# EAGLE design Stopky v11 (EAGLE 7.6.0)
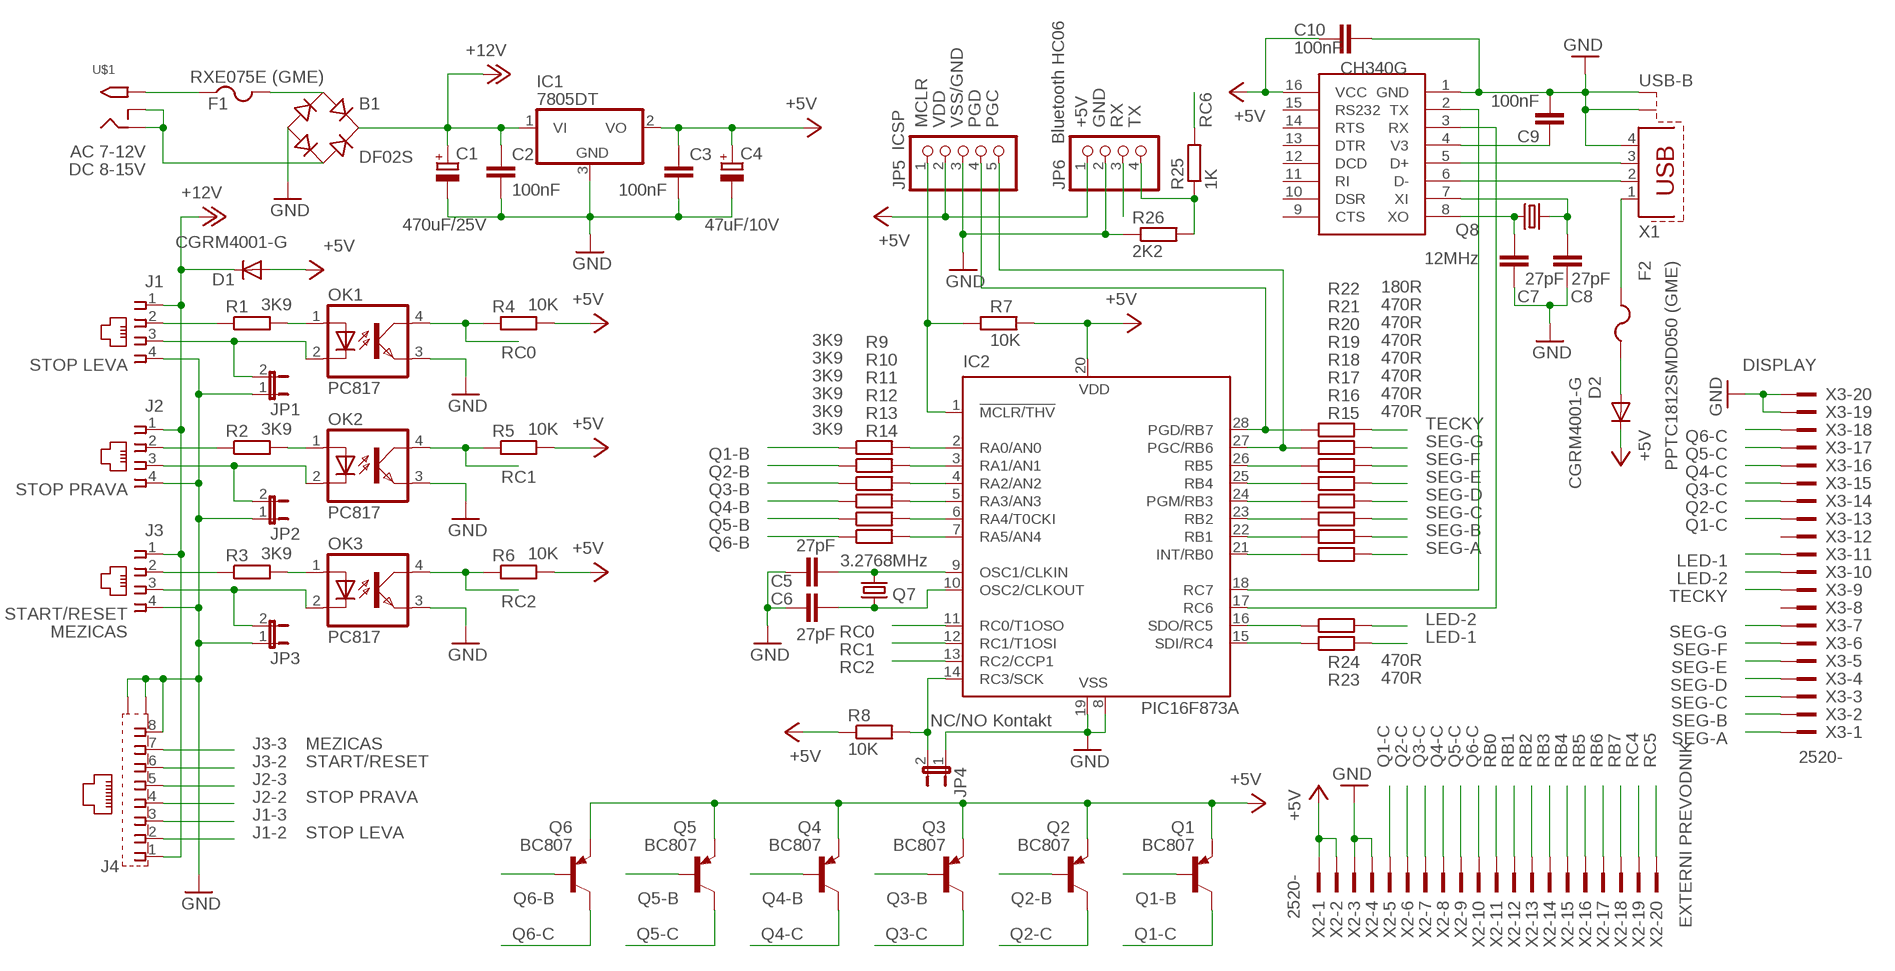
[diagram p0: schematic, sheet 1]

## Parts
B1  DF02S  [DFS]
C1  470uF/25V  CPOL-EUE3.5-10  [E3,5-10]
C2  100nF  C-EUC1206  [C1206]
C3  100nF  C-EUC1206  [C1206]
C4  47uF/10V  CPOL-EUSMCC  [SMC_C]
C5  27pF  C-EUC1206  [C1206]
C6  27pF  C-EUC1206  [C1206]
C7  27pF  C-EUC1206  [C1206]
C8  27pF  C-EUC1206  [C1206]
C9  100nF  C-EUC1206  [C1206]
C10  100nF  C-EUC1206  [C1206]
D1  CGRM4001-G  [SOD-123_MINI-SMA]
D2  CGRM4001-G  [SOD-123_MINI-SMA]
F1  RXE075E (GME)  PTCFUSE-1812  [1812]
F2  PPTC1812SMD050 (GME)  PTCFUSE-1812  [1812]
IC1  7805DT  [TO252]
IC2  PIC16F873A  PIC16873SO  [SO28W]
IC3  CH340G  [SOIC16]
J1  215875-3  [215875-3]
J2  215875-3  [215875-3]
J3  215875-3  [215875-3]
J4  555153-1  [555153-1]
JP1  JP1E  [JP1]
JP2  JP1E  [JP1]
JP3  JP1E  [JP1]
JP4  JP1E  [JP1]
JP5  PINHD-1X5  [1X05]
JP6  PINHD-1X4  [1X04]
OK1  PC817  SFH618A-3X007  [SMD4-7]
OK2  PC817  SFH618A-3X007  [SMD4-7]
OK3  PC817  SFH618A-3X007  [SMD4-7]
Q1  BC807  BC807-16SMD  [SOT23-BEC]
Q2  BC807  BC807-16SMD  [SOT23-BEC]
Q3  BC807  BC807-16SMD  [SOT23-BEC]
Q4  BC807  BC807-16SMD  [SOT23-BEC]
Q5  BC807  BC807-16SMD  [SOT23-BEC]
Q6  BC807  BC807-16SMD  [SOT23-BEC]
Q7  3.2768MHz  CRYSTALSM49  [SM49]
Q8  12MHz  CRYSTALSM49  [SM49]
R1  3K9  R-EU_R1206  [R1206]
R2  3K9  R-EU_R1206  [R1206]
R3  3K9  R-EU_R1206  [R1206]
R4  10K  R-EU_R1206  [R1206]
R5  10K  R-EU_R1206  [R1206]
R6  10K  R-EU_R1206  [R1206]
R7  10K  R-EU_R1206  [R1206]
R8  10K  R-EU_R1206  [R1206]
R9  3K9  R-EU_R1206  [R1206]
R10  3K9  R-EU_R1206  [R1206]
R11  3K9  R-EU_R1206  [R1206]
R12  3K9  R-EU_R1206  [R1206]
R13  3K9  R-EU_R1206  [R1206]
R14  3K9  R-EU_R1206  [R1206]
R15  470R  R-EU_R1206  [R1206]
R16  470R  R-EU_R1206  [R1206]
R17  470R  R-EU_R1206  [R1206]
R18  470R  R-EU_R1206  [R1206]
R19  470R  R-EU_R1206  [R1206]
R20  470R  R-EU_R1206  [R1206]
R21  470R  R-EU_R1206  [R1206]
R22  180R  R-EU_R1206  [R1206]
R23  470R  R-EU_R1206  [R1206]
R24  470R  R-EU_R1206  [R1206]
R25  1K  R-EU_R1206  [R1206]
R26  2K2  R-EU_R1206  [R1206]
U$1  2.1MMJACKTHM  [PJ-102A]
X1  USB-B  PN61729-S  [PN61729-S]
X2  2520-  [PAK100/2500-20]
X3  2520-  [PAK100/2500-20]

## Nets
+5V: C3.1 C4.+ C10.2 D1.A D2.C IC1.2(VO) IC2.20(VDD) IC3.16(VCC) JP5.2 JP6.1 Q1.E Q2.E Q3.E Q4.E Q5.E Q6.E R4.2 R5.2 R6.2 R7.2 R8.1 X2.1 X2.2
+12V: B1.+ C1.+ C2.1 D1.C IC1.1(VI) J1.1 J2.1 J3.1 J4.1
GND: B1.- C1.- C2.2 C3.2 C4.- C5.1 C6.1 C7.1 C8.1 C9.1 C10.1 IC1.3(GND) IC2.8(VSS) IC2.19(VSS) IC3.1(GND) J1.4 J2.4 J3.4 J4.8 J4.G1(S1) J4.G2(S2) JP1.1 JP2.1 JP3.1 JP4.1 JP5.3 JP6.2 OK1.3(EMIT) OK2.3(EMIT) OK3.3(EMIT) R26.1 X1.4 X1.S1 X1.S2 X2.3 X2.4 X3.19 X3.20
J1-2: J1.2 J4.2 R1.1
J1-3: J1.3 J4.3 JP1.2 OK1.2(C)
J2-2: J2.2 J4.4 R2.1
J2-3: J2.3 J4.5 JP2.2 OK2.2(C)
J3-2: J3.2 J4.6 R3.1
J3-3: J3.3 J4.7 JP3.2 OK3.2(C)
LED-1: R23.2 X3.11
LED-2: R24.2 X3.10
N$1: B1.AC2 U$1.RING U$1.RING_SW
N$2: F1.1 U$1.TIP
N$3: B1.AC1 F1.2
N$4: OK1.1(A) R1.2
N$5: OK2.1(A) R2.2
N$6: OK3.1(A) R3.2
N$7: IC2.14(RC3/SCK) JP4.2 R8.2
N$8: IC2.2(RA0/AN0) R9.2
N$9: IC2.3(RA1/AN1) R10.2
N$10: IC2.4(RA2/AN2) R11.2
N$11: IC2.1(!MCLR/THV) JP5.1 R7.1
N$12: C5.2 IC2.9(OSC1/CLKIN) Q7.2
N$13: C6.2 IC2.10(OSC2/CLKOUT) Q7.1
N$14: IC2.5(RA3/AN3) R12.2
N$15: IC2.6(RA4/T0CKI) R13.2
N$16: IC2.7(RA5/AN4) R14.2
N$17: IC3.6(D-) X1.2
N$18: IC3.5(D+) X1.3
N$26: F2.2 X1.1
N$29: C8.2 IC3.7(XI) Q8.1
N$30: C7.2 IC3.8(XO) Q8.2
N$32: C9.2 IC3.4(V3)
N$38: D2.A F2.1
N$41: JP6.4 R25.1 R26.2
Q1-B: Q1.B R9.1
Q1-C: Q1.C X2.5 X3.13
Q2-B: Q2.B R10.1
Q2-C: Q2.C X2.6 X3.14
Q3-B: Q3.B R11.1
Q3-C: Q3.C X2.7 X3.15
Q4-B: Q4.B R12.1
Q4-C: Q4.C X2.8 X3.16
Q5-B: Q5.B R13.1
Q5-C: Q5.C X2.9 X3.17
Q6-B: Q6.B R14.1
Q6-C: Q6.C X2.10 X3.18
RB0: IC2.21(INT/RB0) R15.1 X2.11
RB1: IC2.22(RB1) R16.1 X2.12
RB2: IC2.23(RB2) R17.1 X2.13
RB3: IC2.24(PGM/RB3) R18.1 X2.14
RB4: IC2.25(RB4) R19.1 X2.15
RB5: IC2.26(RB5) R20.1 X2.16
RB6: IC2.27(PGC/RB6) JP5.5 R21.1 X2.17
RB7: IC2.28(PGD/RB7) JP5.4 R22.1 X2.18
RC0: IC2.11(RC0/T1OSO) OK1.4(COL) R4.1
RC1: IC2.12(RC1/T1OSI) OK2.4(COL) R5.1
RC2: IC2.13(RC2/CCP1) OK3.4(COL) R6.1
RC4: IC2.15(SDI/RC4) R23.1 X2.19
RC5: IC2.16(SDO/RC5) R24.1 X2.20
RC6: IC2.17(RC6) IC3.3(RX) R25.2
RC7: IC2.18(RC7) IC3.2(TX) JP6.3
SEG-A: R15.2 X3.1
SEG-B: R16.2 X3.2
SEG-C: R17.2 X3.3
SEG-D: R18.2 X3.4
SEG-E: R19.2 X3.5
SEG-F: R20.2 X3.6
SEG-G: R21.2 X3.7
TECKY: R22.2 X3.9
Unconnected: IC3.9(CTS) IC3.10(DSR) IC3.11(RI) IC3.12(DCD) IC3.13(DTR) IC3.14(RTS) IC3.15(RS232) X3.8 X3.12

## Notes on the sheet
- Bluetooth HC06
- ICSP
- MCLR | VDD | VSS/GND | PGD | PGC | +5V | GND | RX | TX | RC6
- AC 7-12V
- DC 8-15V
- STOP LEVA | RC0 | DISPLAY
- TECKY | Q6-C
- Q1-B | SEG-G | Q5-C
- Q2-B | SEG-F | Q4-C
- STOP PRAVA | RC1 | Q3-B | SEG-E | Q3-C
- Q4-B | SEG-D | Q2-C
- Q5-B | SEG-C | Q1-C
- Q6-B | SEG-B
- SEG-A | LED-1
- LED-2
- TECKY
- START/RESET | RC2
- MEZICAS | RC0 | LED-2 | SEG-G
- RC1 | LED-1 | SEG-F
- RC2 | SEG-E
- SEG-D
- SEG-C
- NC/NO Kontakt | SEG-B
- SEG-A
- J3-3 | MEZICAS
- J3-2 | START/RESET | Q1-C | Q2-C | Q3-C | Q4-C | Q5-C | Q6-C | RB0 | RB1 | RB2 | RB3 | RB4 | RB5 | RB6 | RB7 | RC4 | RC5
- J2-3
- J2-2 | STOP PRAVA
- J1-3
- J1-2 | STOP LEVA
- Q6-B | Q5-B | Q4-B | Q3-B | Q2-B | Q1-B
- Q6-C | Q5-C | Q4-C | Q3-C | Q2-C | Q1-C | EXTERNI PREVODNIK

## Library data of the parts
B1 = rectifier:DF*S: Surface Mount Glass Passivated Bridge Rectifiers Source: Source: Comchip Bridge Rectifiers DF005S-G thru DF10S-G.pdf
C1 C4 = rcl:CPOL-EU: POLARIZED CAPACITOR, European symbol
C2 C3 C5-C10 = rcl:C-EU: CAPACITOR, European symbol
D1 D2 = diode:CGRM400*-G: Molded plasitc,JEDEC SOD-123/Mini SMA
F1 F2 = adafruit:PTCFUSE: PTC fuses, resettable thermistors
IC1 = adafruit:78*: Positive VOLTAGE REGULATOR Added bigger pads to the TO-92 package
IC2 = microchip-6:PIC16*873: MICROCONTROLLER flash type
IC3 = ch340g:CH340G
J1-J3 = con-amp:215875-3: AMP connector
J4 = con-amp:555153-1: AMP connector
JP1-JP4 = jumper:JP1E: JUMPER
JP5 = pinhead:PINHD-1X5: PIN HEADER
JP6 = pinhead:PINHD-1X4: PIN HEADER
OK1-OK3 = optocoupler:SFH618?*: Optocoupler, Phototransistor Output, Low Input Current Source: Data sheet; OC_FARNELL: unknown; OC_NEWARK: unknown
Q1-Q6 = transistor-pnp:BC807*: PNP Transistror
Q7 Q8 = adafruit:CRYSTAL: CRYSTAL; OC_FARNELL: unknown; OC_NEWARK: unknown
R1-R26 = rcl:R-EU_: RESISTOR, European symbol
U$1 = adafruit:2.1MMJACK: 2.1mm x 5.5mm THM DC jack with internal switch. Digikey part #PJ-102A, 4UCON part #05537 2.1mm x 5.5mm SMT DC jack with internal switch. Digikey part #PJ-002A-SMT, 4UCON part #03267 By microbuilder.eu & adafruit.com
X1 = con-berg:PN61729-S: BERG USB connector; OC_FARNELL: unknown; OC_NEWARK: unknown
X2 X3 = con-3m:2520-: 3M (TM) Pak 100 4-Wall Header Source: 3M; OC_FARNELL: unknown; OC_NEWARK: unknown

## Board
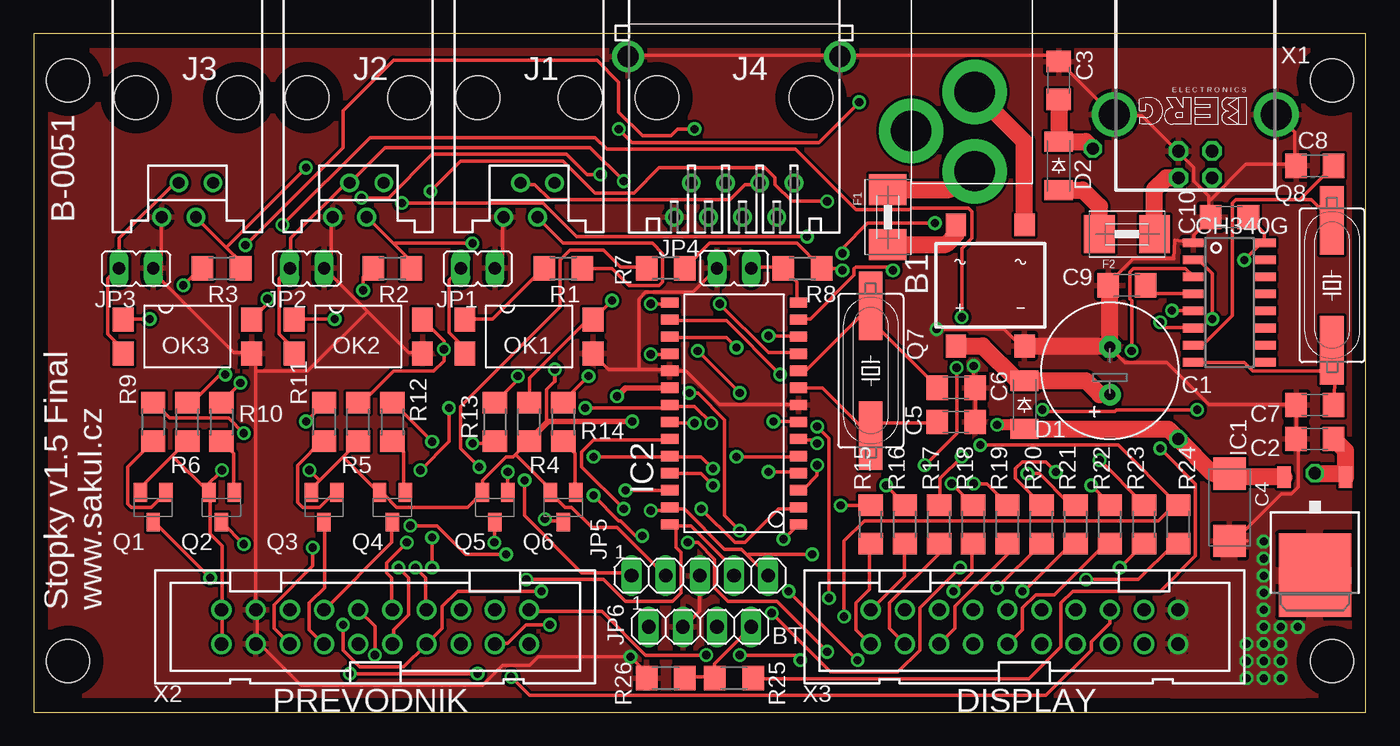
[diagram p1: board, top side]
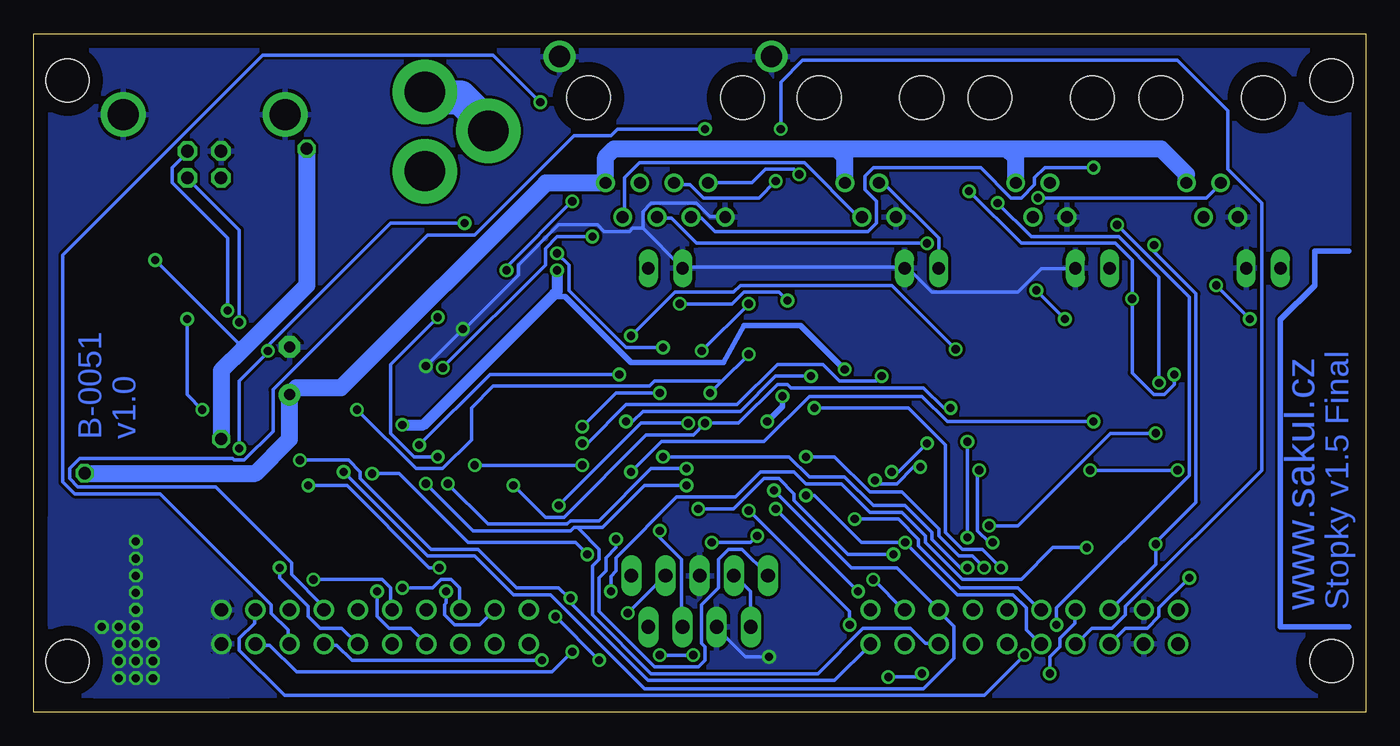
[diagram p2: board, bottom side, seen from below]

Size 99.04 x 50.47 mm. Coordinates in mm from the lower left corner, seen from the top.
Outline: 0,0 99.04,0 99.04,50.47 0,50.47 0,0
Copper layers (1*16): Top 0.035mm / dielectric 1.5mm / Bottom 0.035mm
Design rules "default": minimum track width 10mil, minimum drill 24mil, track to track 8mil, track to pad 8mil, pad to pad 8mil, via to via 8mil, smd to smd 8mil, copper to edge 40mil, drill to drill 8mil, minimum pad ring 10mil, minimum via ring 8mil, stop-mask expansion 4mil, vias tented up to drill 0mil, thermal gap 10mil
Holes 3.2 mm at 2.54,46.99 96.52,46.99 2.54,3.81 96.52,3.81

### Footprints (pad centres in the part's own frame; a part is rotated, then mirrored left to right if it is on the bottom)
DFS = smd 1.5 x 1.7: + -2.55,-4.5; - 2.55,-4.5; AC1 -2.55,4.5; AC2 2.55,4.5
E3,5-10 = drill 0.813 pad 1.6: + -1.778,0 | drill 0.813 pad 1.6 octagon: - 1.778,0
C1206 = smd 1.6 x 1.8: 1 -1.4,0; 2 1.4,0
SMC_C = smd 2.4 x 2.4: + -2.5,0; - 2.5,0
SOD-123_MINI-SMA = smd 1.5 x 2.1: A 1.8,0; C -1.8,0
1812 = smd 2.286 x 2.794: 1 -2.046,0; 2 2.046,0
TO252 = smd 1 x 1.6: 1 -2.28,-4.8; 2 2.28,-4.8 | smd 5.4 x 6.2: 3 0,2.5
SO28W = smd 0.762 x 1.27: 1 -7.62,-4.78; 2 -6.35,-4.78; 3 -5.08,-4.78; 4 -3.81,-4.78; 5 -2.54,-4.78; 6 -1.27,-4.78; 7 0,-4.78; 8 1.27,-4.78; 9 2.54,-4.78; 10 3.81,-4.78; 11 5.08,-4.78; 12 6.35,-4.78; 13 7.62,-4.78; 14 8.89,-4.78; 15 8.89,4.78; 16 7.62,4.78; 17 6.35,4.78; 18 5.08,4.78; 19 3.81,4.78; 20 2.54,4.78; 21 1.27,4.78; 22 0,4.78; 23 -1.27,4.78; 24 -2.54,4.78; 25 -3.81,4.78; 26 -5.08,4.78; 27 -6.35,4.78; 28 -7.62,4.78
SOIC16 = smd 0.635 x 1.524: 1 -4.445,-2.695; 2 -3.175,-2.695; 3 -1.905,-2.695; 4 -0.635,-2.695; 5 0.635,-2.695; 6 1.905,-2.695; 7 3.175,-2.695; 8 4.445,-2.695; 9 4.445,2.695; 10 3.175,2.695; 11 1.905,2.695; 12 0.635,2.695; 13 -0.635,2.695; 14 -1.905,2.695; 15 -3.175,2.695; 16 -4.445,2.695
215875-3 = drill 0.889: 1 -1.905,6.35; 2 -0.635,8.89; 3 0.635,6.35; 4 1.905,8.89 | hole 3.251: -3.81,0; 3.81,0
555153-1 = drill 0.889: 1 -4.445,6.35; 2 -3.175,8.89; 3 -1.905,6.35; 4 -0.635,8.89; 5 0.635,6.35; 6 1.905,8.89; 7 3.175,6.35; 8 4.445,8.89 | drill 1.575 pad 2.184: G1 -7.874,-3.048; G2 7.874,-3.048 | hole 3.251: -5.715,0; 5.715,0
JP1 = drill 0.914 long: 1 0,-1.27; 2 0,1.27
1X05 = drill 1.016 long: 1 -5.08,0; 2 -2.54,0; 3 0,0; 4 2.54,0; 5 5.08,0
1X04 = drill 1.016 long: 1 -3.81,0; 2 -1.27,0; 3 1.27,0; 4 3.81,0
SMD4-7 = smd 1.78 x 1.55: 1 -1.27,-4.77; 2 1.27,-4.77; 3 1.27,4.77; 4 -1.27,4.77
SOT23-BEC = smd 1 x 1.4: B -0.95,-1.1; C 0,1.1; E 0.95,-1.1
SM49 = smd 5.08 x 1.778: 1 -4.826,0; 2 4.826,0
R1206 = smd 1.6 x 1.803: 1 -1.422,0; 2 1.422,0
PJ-102A = drill 3 pad 4.8: RING 0.1,-3.39; RING_SW -4.6,-6.29; TIP 0.1,-9.29
PN61729-S = drill 0.95 octagon: 1 1.25,4.71; 2 -1.25,4.71; 3 -1.25,2.71; 4 1.25,2.71 | drill 2.3 pad 2.9: S1 -6.02,0; S2 6.02,0
PAK100/2500-20 = drill 1 pad 1.422: 1 -11.43,-1.27; 2 -11.43,1.27; 3 -8.89,-1.27; 4 -8.89,1.27; 5 -6.35,-1.27; 6 -6.35,1.27; 7 -3.81,-1.27; 8 -3.81,1.27; 9 -1.27,-1.27; 10 -1.27,1.27; 11 1.27,-1.27; 12 1.27,1.27; 13 3.81,-1.27; 14 3.81,1.27; 15 6.35,-1.27; 16 6.35,1.27; 17 8.89,-1.27; 18 8.89,1.27; 19 11.43,-1.27; 20 11.43,1.27

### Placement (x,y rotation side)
B1  71.12,31.75 0 top
C1  80.01,25.4 90 top
C2  95.25,20.32 180 top
C3  76.2,46.99 90 top
C4  88.9,15.24 270 top
C5  68.58,21.59 180 top
C6  68.58,24.13 180 top
C7  95.25,22.86 0 top
C8  95.25,40.64 0 top
C9  81.28,31.75 0 top
C10  88.9,36.83 0 top
D1  73.66,22.86 270 top
D2  76.2,40.64 270 top
F1  63.5,36.83 270 top
F2  81.28,35.56 0 top
IC1  95.25,12.7 180 top
IC2  52.07,21.59 90 top
IC3  88.9,30.48 270 top
J1  36.83,45.72 180 top
J2  24.13,45.72 180 top
J3  11.43,45.72 180 top
J4  52.07,45.72 180 top
JP1  33.02,33.02 90 top
JP2  20.32,33.02 90 top
JP3  7.62,33.02 90 top
JP4  52.07,33.02 270 top
JP5  49.53,10.16 0 top
JP6  49.53,6.35 0 top
OK1  36.83,27.94 270 top
OK2  24.13,27.94 270 top
OK3  11.43,27.94 270 top
Q1  8.89,15.24 180 top
Q2  13.97,15.24 180 top
Q3  21.59,15.24 180 top
Q4  26.67,15.24 180 top
Q5  34.29,15.24 180 top
Q6  39.37,15.24 180 top
Q7  62.23,25.4 270 top
Q8  96.52,31.75 270 top
R1  39.37,33.02 180 top
R2  26.67,33.02 180 top
R3  13.97,33.02 180 top
R4  36.83,21.59 270 top
R5  24.13,21.59 270 top
R6  11.43,21.59 270 top
R7  46.99,33.02 0 top
R8  57.15,33.02 180 top
R9  8.89,21.59 90 top
R10  13.97,21.59 90 top
R11  21.59,21.59 90 top
R12  26.67,21.59 90 top
R13  34.29,21.59 90 top
R14  39.37,21.59 90 top
R15  62.23,13.97 270 top
R16  64.77,13.97 270 top
R17  67.31,13.97 270 top
R18  69.85,13.97 270 top
R19  72.39,13.97 270 top
R20  74.93,13.97 270 top
R21  77.47,13.97 270 top
R22  80.01,13.97 270 top
R23  82.55,13.97 270 top
R24  85.09,13.97 270 top
R25  52.07,2.54 0 top
R26  46.99,2.54 0 top
U$1  69.85,49.53 0 top
X1  86.36,44.45 180 top
X2  25.4,6.35 0 top
X3  73.66,6.35 0 top

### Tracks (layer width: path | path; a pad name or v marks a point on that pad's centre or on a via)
+5V  (via drill 0.61, 0.9)
  Top 0.254: R7.2 48.5,33.12 50.25,34.88 56.75,34.88 58.5,33.12 R8.1 58.62,33 60,33 v60.12,32.88 | C10.2 90.38,36.75 91.5,35.62 91.5,35 IC3.16 91.38,35 v90,33.62 | 73.12,21.38 D1.A | X2.1 14,5.12 14,7.5 X2.2 14,7.75 14,12.38 13.12,13.25 13.12,16.25 Q2.E | 10.31,19.06 11.38,20.12 R6.2 | 10.31,19.06 8,16.75 8,16.38 Q1.E | 10.31,19.06 13,16.38 Q2.E | 23,19 24.12,20.12 R5.2 | 23,19 21.25,17.25 | 21.25,17.25 20.75,16.75 20.75,16.38 Q3.E | 23,19 25.62,16.38 Q4.E 25.75,16.25 26,16.25 27,15.25 32.25,15.25 Q5.E 33.38,16.38 33.38,17.25 35.12,19 35.62,19 35.81,19.19 | 47.25,24.12 IC2.20 | 36.88,20.25 R4.2 36.75,20.12 35.81,19.19 | 35.81,19.19 38.38,16.62 38.38,16.38 Q6.E 38.5,16.25 39.5,15.25 40,15.25 41.5,13.75 43.38,13.75 46.88,10.25 JP5.2 | v14,18 12.75,16.75 Q2.E | 21.25,17.25 v20.5,18 | 38.75,24.62 38.12,24 38.12,21.62 38.25,21.62
  Top 0.305: 38.75,24.62 v38.75,25.5
  Top 0.406: 47.25,24.12 44,24.12 v43.38,23.5 | v44.5,21.62 38.25,21.62 36.88,20.25
  Top 0.813: 73.12,21.38 v71.62,21.38
  Top 1.27: C3.1 D2.C 78.21,42.44 v78.74,41.91 | IC1.2 89.14,17.5 C4.+ 88.86,17.78 87.63,17.78 v85.09,20.32 84.35,21.06 D1.A
  Bottom 0.254: 83.43,27.06 v90,33.62 | JP6.1 45.75,6.38 45.75,9 46.88,10.12 JP5.2 | v20.5,18 v14,18 | 60.13,30.92 60.33,31.11
  Bottom 0.406: v43.38,23.5 43.38,22.75 v44.5,21.62 | v38.75,25.5 42.02,28.77 46.25,28.77 47.75,26 54.62,26 59.54,30.92 60.13,30.92
  Bottom 0.813: v71.62,21.38 70.06,21.38 60.33,31.11 60.12,31.32 v60.12,32.88
  Bottom 1.27: v78.74,41.91 78.74,31.75 83.43,27.06 85.09,25.4 v85.09,20.32
+12V  (via drill 0.9)
  Top 1.27: B1.+ 70.54,27.25 73.13,24.66 D1.C 78.21,24.66 79.25,23.62 C1.+ | C2.1 97.53,19.44 IC1.1 97.25,17.78 v95.25,17.78
  Bottom 1.27: 39.37,41.91 55.88,41.91 56.52,41.27 J4.1 60.96,39.37 76.2,24.13 79.5,24.13 C1.+ 80.01,20.32 82.55,17.78 v95.25,17.78 | 39.37,41.91 26.67,41.91 | 26.67,41.91 15.24,41.91 13.34,40.01 J3.1 | J2.1 26.04,41.27 26.67,41.91 | J1.1 38.73,41.27 39.37,41.91
GND  (via drill 0.6, 0.61)
  Top 0.254: 45,25.5 42.75,25.5 41.62,26.62 OK1.3 | 45,25.5 47.25,25.5 IC2.19 47.38,25.38 48.5,25.38 51,22.88 56.75,22.88 IC2.8 | J1.4 34.88,36.75 34.88,33.62 34.38,33.12 JP1.1 | 45,25.5 45,30.75 45.5,31.25 49,31.25 50.75,33 JP4.1 | 24.81,29.81 21.62,33 JP2.1 22.12,32.62 22.12,36.75 J2.4 | 24.81,29.81 27.88,26.75 28.88,26.75 OK2.3 | R26.1 45.5,2.62 45.5,3 v44.38,4.12 37.5,4.12 36.88,3.5 34.88,3.5 33.38,2 19.88,2 16.75,5.12 X2.3 16.62,5.12 16.62,7.5 X2.4 16.5,25.38 | JP5.3 49.5,10.12 49.5,7.5 48.38,6.38 JP6.2 | J3.4 9.5,36.75 9.5,32.25 JP3.1 9,33 9,32.62 14.88,26.75 16.12,26.75 OK3.3 16.25,26.62 16.5,26.38 16.5,25.38 | 24.81,29.81 20.38,25.38 16.5,25.38 | J4.G2 44.25,48.88 59.88,48.88 J4.G1 60,48.88 75.75,48.88 76.12,48.5 C3.2 76.25,48.38 80.25,44.38 X1.S2 80.38,44.38 82.38,44.38 85,41.75 X1.4 85.12,41.62 86.25,40.5 86.25,39.5 87.38,38.38 87.38,38.12 | 90.21,12.74 89.62,12.75 89,12.75 C4.- 89.62,12.88 89.62,13.12 92.75,16.25 93.5,16.25 94,16.75 94,20.38 C2.2 93.88,20.38 93.88,22.75 C7.1 93.75,22.88 87.38,22.88 84.25,26 81.12,26 80.38,26.75 C1.- | X1.S1 92.5,44.38 93.75,43.12 93.75,40.75 C8.1 93.62,40.75 90.12,40.75 87.5,38.12 87.38,38.12 | C5.1 70,21.62 70,24.12 C6.1 69.88,24.25 v69.88,25.75 | v67.12,28.5 72.12,28.5 73.12,27.5 B1.- | 87.38,38.12 87.38,36.88 C10.1 87.5,36.75 86.25,35.5 86.25,35 IC3.1 84.86,35.12 84.75,33.75 81.75,33.75 80.25,32.25 C9.1
  Top 1.27: B1.- 79.94,27.25 C1.- 80.01,31.62 C9.1
  Bottom 0.254: 53.75,36 53.75,37.25 53.12,37.88 49.75,37.88 48.75,36.88 47.62,36.88 J4.8 | 53.75,36 50.88,33.12 JP4.1 50.75,33.12 34.38,33.12 JP1.1 34.25,33 34,33 32.25,31.25 25.88,31.25 24.12,33 21.62,33 JP2.1 | v44.38,4.12 46.12,4.12 48.25,6.25 JP6.2 | v69.88,25.75 v67.12,28.5 67,28.5 63,32.5 63,33.25 60,36.25 57.12,36.25 56.62,35.75 54.75,35.75 54.5,36 53.75,36
  other vias: 91.44,12.7 91.44,11.43 91.44,10.16 91.44,8.89 91.44,7.62 91.44,6.35 92.71,6.35 93.98,6.35 91.44,5.08 91.44,2.54 90.17,2.54 92.71,5.08 91.44,3.81 92.71,3.81 92.71,2.54 90.17,3.81 90.17,5.08
  pour Bottom: 97.79,13.97 88.9,13.97 85.09,10.16 85.09,1.27 97.79,1.27
  pour Top: 97.79,13.97 91.44,13.97 85.09,7.62 85.09,1.27 97.79,1.27
  pour Bottom: 1.27,49.53 97.79,49.53 97.79,1.27 1.27,1.27
  pour Top: 1.27,49.53 97.79,49.53 97.79,1.27 1.27,1.27
J1-2
  Top 0.254: R1.1 40.88,33 43,33 44.25,31.75 46.5,31.75 46.75,32 46.75,34.12 46,34.88 39.38,34.88 37.5,36.75 J1.2
  Bottom 0.254: J4.2 55.12,36.88 55.12,39.75 54,40.88 41.75,40.88 37.75,36.88 37.5,36.88 J1.2
J1-3
  Top 0.254: OK1.2 32,26.75 32,27.12 30.88,28.25 30.88,32.12 31.75,33 JP1.2 | J4.3 53.88,39.25 52.88,39.25 51.75,38.12 38.38,38.12 37.25,39.25 36.25,39.25 J1.3
  Bottom 0.254: JP1.2 31.75,35.25 35.75,39.25 36.12,39.25 J1.3
J2-2  (via drill 0.61)
  Top 0.254: 26.81,34.81 24.88,36.75 J2.2 | 26.81,34.81 28,33.62 28,33.12 R2.1 | v32.62,34.88 26.88,34.88 26.81,34.81
  Bottom 0.254: v32.62,34.88 49.75,34.88 51.62,36.75 52.62,36.75 J4.4
J2-3  (via drill 0.61)
  Top 0.254: OK2.2 19.25,26.75 19.25,27.12 18.25,28.12 18.25,32.25 19,33 JP2.2 19.12,33.12 19.12,35.25 23.12,39.25 23.38,39.25 J2.3 26.12,42 41.38,42 v43.88,39.5
  Bottom 0.254: v43.88,39.5 45.12,38.25 49.25,38.25 50.25,39.25 51.38,39.25 J4.5
J3-2  (via drill 0.61)
  Top 0.254: 14.31,34.56 12.12,36.75 J3.2 | 14.31,34.56 15.38,33.5 15.38,33.12 R3.1 | 14.31,34.56 v20.25,40.5
  Bottom 0.254: v20.25,40.5 23.88,40.5 24.62,39.75 24.62,39.25 25.62,38.25 26.38,38.25 28.62,40.5 36.62,40.5 37.25,39.88 37.25,38.88 36.38,38 36.38,36.38 37,35.75 48.38,35.75 49.38,36.75 50.12,36.75 J4.6
J3-3  (via drill 0.61)
  Top 0.254: OK3.2 6.62,26.75 6.62,27 5.5,28.12 5.5,32.25 6.25,33 JP3.2 6.38,33.12 6.38,35.25 10.38,39.25 10.75,39.25 J3.3 | v42.12,40 41.12,40 39.62,41.5 29.62,41.5 26.38,38.25 v24.38,38.25
  Bottom 0.254: v42.12,40 42.5,40.38 44.62,40.38 45.62,39.38 48.88,39.38 J4.7 | v24.38,38.25 11.88,38.25 10.88,39.25 J3.3
LED-1  (via drill 0.61)
  Top 0.254: v80.75,10.75 82.5,12.5 R23.2
  Bottom 0.254: v80.75,10.75 80.75,10 78.62,7.88 78.62,7.12 77.75,6.25 76.12,6.25 75,5.12 X3.11
LED-2  (via drill 0.61)
  Top 0.254: v78.25,9.88 82.12,9.88 84.75,12.5 85,12.5 R24.2
  Bottom 0.254: v78.25,9.88 73.12,9.88 72.5,9.25 72.5,7.62 X3.10
N$1
  Top 1.27: B1.AC2 73.67,42.42 U$1.RING
  Bottom 2.54: U$1.RING_SW 65.25,43.66 67.31,45.72 69.53,45.72 U$1.RING
N$2
  Top 1.27: U$1.TIP 69.45,40.24 68.09,38.88 F1.1
N$3
  Top 1.27: F1.2 67.8,34.78 68.58,35.56 B1.AC1
N$4
  Top 0.254: OK1.1 32.12,29.25 34.12,29.25 37.88,33 R1.2
N$5  (via drill 0.61)
  Top 0.254: v22.38,29.25 19.38,29.25 OK2.1 | v24.5,31.38 24.5,32.38 25.12,33 R2.2
  Bottom 0.254: v24.5,31.38 v22.38,29.25
N$6  (via drill 0.61)
  Top 0.254: v8.62,29.25 6.75,29.25 OK3.1 | v11.12,31.75 12.5,33.12 R3.2
  Bottom 0.254: v11.12,31.75 v8.62,29.25
N$7
  Top 0.254: IC2.14 56.75,30.5 56.75,32 55.75,33 R8.2 55.62,33.12 53.38,33.12 JP4.2
N$8  (via drill 0.61)
  Top 0.254: v49.62,15.12 52.12,12.62 52.88,12.62 55.38,15.12 56.75,15.12 IC2.2 | v35.12,11.75 32.12,11.75 30,13.88 v28,13.88 | v15.62,20.75 14.5,21.88 10.12,21.88 9,23 R9.2
  Bottom 0.254: v49.62,15.12 47,15.12 44.75,17.38 43.62,17.38 42.5,16.25 42.5,15.75 38.5,11.75 v35.12,11.75 | v28,13.88 25.88,13.88 19,20.75 v15.62,20.75
N$9  (via drill 0.61)
  Top 0.254: v58.25,18.38 58.25,17.62 57.25,16.62 56.88,16.62 IC2.3 | v66.25,18.38 68.62,20.75 v68.62,25.62 | v57.5,35.38 40.38,35.38 37.88,37.88 v27.38,37.88 | v15.38,24.5 14,23.12 R10.2
  Bottom 0.254: v66.25,18.38 v58.25,18.38 | v68.62,25.62 61,33.25 61,34.5 60.12,35.38 v57.5,35.38 | v27.38,37.88 24.88,35.38 18.38,35.38 15.38,32.38 v15.38,24.5
N$10  (via drill 0.61)
  Top 0.254: v54.62,17.88 56.75,17.88 IC2.4 | v20.25,21.62 21.62,23 R11.2
  Bottom 0.254: v54.62,17.88 52.38,20.12 44.75,20.12 41.38,23.5 33,23.5 31.12,21.62 v20.25,21.62
N$11  (via drill 0.61)
  Top 0.254: v55.75,12.88 56.75,13.88 IC2.1 | v33.12,18.25 31.75,19.62 31.75,22.75 39.12,30.12 39.12,33.62 39.88,34.38 42.38,34.38 43.62,33.12 45.5,33.12 R7.1 | v36.5,17.25 36.5,14.62 40.75,10.38 44.25,10.38 44.38,10.25 JP5.1
  Bottom 0.254: v55.75,12.88 55.75,12.25 56.5,11.5 56.5,10.5 57,10 57,7.5 52.88,3.38 49.62,3.38 49.12,3.88 49.12,4.88 49.38,5.12 49.38,8 48.12,9.25 48.12,11.38 47.38,12.12 46.38,12.12 44.5,10.25 JP5.1 | v33.12,18.25 33.62,18.25 34.88,17 36.25,17 v36.5,17.25
N$12
  Top 0.254: IC2.9 56.88,24.12 58.62,24.12 62.12,20.62 Q7.2 61.38,21.5 67.12,21.5 C5.2
N$13
  Top 0.254: IC2.10 56.88,25.5 57.5,25.5 62.12,30.12 Q7.1 61.75,29.62 67.12,24.25 C6.2
N$14  (via drill 0.61)
  Top 0.254: v52.25,19 56.75,19 IC2.5 | v29.62,13 v29.62,10.75 | v29.62,20.12 26.75,23 R12.2
  Bottom 0.254: v52.25,19 42.88,19 41.38,17.5 38.75,17.5 36.62,15.38 34.25,15.38 32.25,13.38 32.25,12.88 30.12,10.75 v29.62,10.75 | v29.62,20.12 v29.62,13
N$15  (via drill 0.61)
  Top 0.254: v58.25,20 58,20.25 56.88,20.25 IC2.6 | v36,25 36,24.75 34.38,23.12 R13.2
  Bottom 0.254: v58.25,20 57.88,20 55,22.88 46.75,22.88 43.75,25.88 40.38,25.88 39.12,24.62 36.38,24.62 v36,25
N$16  (via drill 0.61)
  Top 0.254: v55,21.62 56.75,21.62 IC2.7 | v41.25,25 39.38,23.12 R14.2
  Bottom 0.254: v55,21.62 54.5,21.62 53.75,22.38 46.5,22.38 43.88,25 v41.25,25
N$17  (via drill 0.61)
  Top 0.254: v83.75,29 84.12,28.62 86.12,28.62 IC3.6
  Bottom 0.254: v83.75,29 83.75,35.88 87.5,39.62 X1.2
N$18  (via drill 0.61)
  Top 0.254: v84.62,29.88 86.12,29.88 IC3.5
  Bottom 0.254: v84.62,29.88 84.62,35.25 88.75,39.38 88.75,40.5 87.62,41.62 X1.3
N$19
  Bottom 0.406: 1.27,6.35 6.35,6.35 6.35,29.21 3.81,31.75 3.81,34.29 1.27,34.29
N$26
  Top 1.27: X1.1 84.19,39.74 83.33,38.88 F2.2
N$29
  Top 0.254: 94.25,38.12 95,38.12 96.5,36.62 Q8.1 | 94.25,38.12 89.38,38.12 89.12,37.88 89.12,29.5 87,27.38 86.25,27.38 IC3.7 | C8.2 96.62,40.62 94.25,38.25 94.25,38.12
N$30
  Top 0.254: 95.52,25.38 96.27,25.38 96.5,26.88 Q8.2 | 95.52,25.38 90.62,25.38 90,26 86.25,26 IC3.8 | C7.2 96.62,22.88 96.79,25.25 95.52,25.38
N$32
  Top 0.254: IC3.4 86.12,31.12 83.38,31.12 82.75,31.75 C9.2
N$38
  Top 1.27: F2.1 79.23,37.61 78,38.84 D2.A
N$41
  Top 0.254: R26.2 48.5,2.62 50.62,2.62 R25.1 50.62,2.75 50.62,3.62 53.25,6.25 JP6.4
Q1-B
  Top 0.254: Q1.B 8.75,15.25 7.25,15.25 7,15.5 7,18.25 8.88,20.12 R9.1
Q1-C  (via drill 0.61)
  Top 0.254: v13.12,10 9,14.12 Q1.C | v56.12,9 v61.25,3.88 | v20.75,12.25 20.75,10.88 17.88,8 17.88,6.25 19,5.12 X2.5
  Bottom 0.254: v13.12,10 15.38,7.75 15.38,7.12 16.25,6.25 17.88,6.25 19,5.12 X2.5 | v61.25,3.88 75.38,3.88 76.5,5 77.38,5 X3.13 | v56.12,9 56.12,10.12 55.75,10.5 55.75,11.5 51.25,16 46.88,16 45,17.88 42.5,17.88 41.62,17 39,17 36.88,14.88 34.5,14.88 32.75,13.12 32.75,12.62 30,9.88 25.62,9.88 23.25,12.25 v20.75,12.25
Q2-B
  Top 0.254: Q2.B 14.88,16.38 14.88,19.25 14,20.12 R10.1
Q2-C  (via drill 0.61)
  Top 0.254: v15.62,12.5 14,14.12 Q2.C | v49.12,43.38 47.88,43.38 47.38,42.88 45.25,42.88 43.5,44.62 43.5,46.88 41.88,48.5 26.75,48.5 23,44.75 23,42 v15.75,34.75
  Bottom 0.254: X2.6 19,7.62 15.62,11 v15.62,12.5 15.62,12.62 12.62,15.62 12.62,31.12 15.75,34.25 v15.75,34.75 | v49.12,43.38 55.62,43.38 56.12,42.88 58.88,42.88 66.25,35.5 69.75,35.5 81.25,24 81.25,20.88 83.38,18.75 84.12,18.75 84.25,18.88 95.62,18.88 96.38,18.12 96.38,17.38 95.75,16.75 85.5,16.75 79.88,11.12 79.88,10.25 77.5,7.88 77.5,7.62 X3.14
Q3-B
  Top 0.254: Q3.B 22.5,16.25 22.25,16.25 21.25,15.25 20,15.25 19.62,15.62 19.62,18.38 21.5,20.25 R11.1
Q3-C  (via drill 0.61)
  Top 0.254: Q3.C 21.62,14.12 21.62,9.25 20.5,8.12 20.5,6.12 21.5,5.12 X2.7 | v61.38,45.38 58.38,42.38 44.5,42.38 v43.5,43.38
  Bottom 0.254: v61.38,45.38 64.88,48.88 82,48.88 96.88,34 96.88,17.12 96,16.25 89.62,16.25 81.38,8 81.38,7.38 80.12,6.12 80.12,5.12 X3.15 | v43.5,43.38 43.5,46.88 41.88,48.5 14,48.5 10.25,44.75 10.25,40.38 7.75,37.88 7.75,18 17.88,7.88 17.88,7.25 18.88,6.25 20.38,6.25 21.5,5.12 X2.7
Q4-B
  Top 0.254: Q4.B 27.5,16.38 27.5,19.38 26.75,20.12 R12.1
Q4-C  (via drill 0.61)
  Top 0.254: Q4.C 26.62,14.12 26.62,12.62 21.62,7.62 X2.8 | v35.5,2.62 36.88,1.25 75.25,1.25 78.62,4.62 78.62,5.25 80,6.62 80,7.5 X3.16 | v23.5,2.88 v33,2.88
  Bottom 0.254: v35.5,2.62 33.25,2.62 v33,2.88 | v23.5,2.88 23.5,4.12 22.75,4.88 22.75,5.5 21.62,6.62 21.62,7.5 X2.8
Q5-B  (via drill 0.61)
  Top 0.254: v35.25,17.88 35.25,16.38 Q5.B | v32.62,20 34.12,20 34.25,20.12 R13.1
  Bottom 0.254: v35.25,17.88 34.75,17.88 v32.62,20
Q5-C  (via drill 0.61)
  Top 0.254: v34.25,12.62 34.25,14.12 Q5.C | v59,4.5 55.25,8.25 51.62,8.25 50.62,9.25 50.62,11.38 49.38,12.62 v48.62,12.62 | v45.25,13.12 44.75,13.12 43.62,14.25 43.5,14.25 v41.62,16.12
  Bottom 0.254: X2.9 24.25,5.12 25.25,6.12 25.25,7.75 26.25,8.75 30.38,8.75 v34.25,12.62 37.5,12.62 41,16.12 v41.62,16.12 | v59,4.5 60.5,3 79.5,3 81.5,5 82.5,5 X3.17 | v48.62,12.62 45.75,12.62 v45.25,13.12
Q6-B
  Top 0.254: Q6.B 40.25,16.38 40.25,19.25 39.38,20.12 R14.1
Q6-C  (via drill 0.61)
  Top 0.254: v38,14.38 38.12,14.25 39.25,14.25 Q6.C | v25.38,4.25 25.38,6.38 X2.10
  Bottom 0.254: v38,14.38 34.75,14.38 33.25,12.88 33.25,12.38 30.12,9.25 25.88,9.25 24.25,7.62 X2.10 | v25.38,4.25 28.38,1.25 80.38,1.25 83.75,4.62 83.75,5.5 82.62,6.62 82.62,7.5 X3.18
RB0  (via drill 0.61)
  Top 0.254: v50.38,21.5 49.12,22.75 47.38,22.75 IC2.21 47.38,22.62 v41,22.62 | v60,15.38 62.12,15.38 R15.1 | v27.12,10.75 27.88,10 27.88,7.25 26.75,6.12 26.75,5.12 X2.11
  Bottom 0.254: v50.38,21.5 53.88,21.5 v60,15.38 | v27.12,10.75 28.5,12.12 30,12.12 31.25,13.38 31.25,19.88 34,22.62 v41,22.62
RB1  (via drill 0.61)
  Top 0.254: v49.12,21.5 47.38,21.5 IC2.22 | v63.38,16.88 64.75,15.5 R16.1 | v27.75,12.62 26.25,11.12 26.25,10.38 26.62,10 26.62,7.62 X2.12 | v28.75,18 30.88,20.12 v30.88,22.62
  Bottom 0.254: v63.38,16.88 61,14.5 59.62,14.5 53.5,20.62 50,20.62 v49.12,21.5 46.62,21.5 43.75,24.38 43,24.38 42.75,24.12 32.88,24.12 31.38,22.62 v30.88,22.62 | v27.75,12.62 28,12.62 28.88,13.5 28.88,17.88 v28.75,18
RB2  (via drill 0.61)
  Top 0.254: v43.88,15.12 40.75,18.25 40.75,19.38 41.62,20.25 47.25,20.25 IC2.23 | v37.75,9 31.5,9 30.38,7.88 30.38,6.25 29.25,5.12 X2.13 29.12,5 27.5,3.38 24.25,3.38 23,4.62 v23,6.5 | v69,19 67.38,17.38 67.38,15.5 R17.1 | v69,29.38 69,34.5 69.75,35.25 69.75,37.25 69.5,37.5 65.25,37.5 65.12,37.38 61.12,37.38 56.62,41.88 42.62,41.88 41.75,42.75 25,42.75 v18.5,36.25
  Bottom 0.254: v37.75,9 v43.88,15.12 | v69,19 70.75,19 72.5,20.75 72.5,25.88 v69,29.38 | v18.5,36.25 13.12,30.88 13.12,17.62 23,7.75 v23,6.5
RB3  (via drill 0.61)
  Top 0.254: v50.5,18.12 49.62,19 47.38,19 IC2.24 47.25,19 v41.62,19 | v68.25,17 69.75,15.5 R18.1 | v28.38,10.75 29.12,10 29.12,7.62 X2.14
  Bottom 0.254: v50.5,18.12 53.12,18.12 57,14.25 59.12,14.25 59.38,14 65.25,14 v68.25,17 | v28.38,10.75 29.25,11.62 30.25,11.62 31.75,13.12 31.75,13.62 34.5,16.38 36.88,16.38 39.5,19 v41.62,19
RB4  (via drill 0.61)
  Top 0.254: v50.5,16.88 49.62,17.75 47.38,17.75 IC2.25 | v69.88,17 70.88,17 72.38,15.5 R19.1
  Bottom 0.254: v50.5,16.88 53.62,16.88 56.75,13.75 58.5,13.75 | 58.5,13.75 58.88,13.75 59.12,13.5 66.38,13.5 v69.88,17 | X2.15 31.75,5.12 32.75,5.12 33.88,6.25 37.38,6.25 40.75,2.88 53.12,2.88 57.5,7.25 57.5,10.88 57,11.38 57,12.12 58.5,13.62 58.5,13.75
RB5  (via drill 0.61)
  Top 0.254: v44,16.5 47.25,16.5 IC2.26 | v76,17.88 75.25,18.62 73.5,18.62 73,18.12 73,17.38 74.88,15.5 R20.1
  Bottom 0.254: v44,16.5 38.25,10.75 34.88,10.75 X2.16 31.75,7.5 30.62,6.38 30.62,4 32.88,1.75 53.62,1.75 60.62,8.75 63.38,8.75 66.25,11.62 69.75,11.62 v76,17.88
RB6  (via drill 0.61)
  Top 0.254: 53.06,11.69 54.5,10.25 JP5.5 | 53.06,11.69 52.62,12.12 51.38,12.12 48.38,15.12 47.38,15.12 IC2.27 47.38,15 v45.88,15 | v73.88,17.75 74.75,17.75 77,15.5 77.38,15.5 R21.1 | v57.88,11.75 53.12,11.75 53.06,11.69 | v38.38,6.5 36.62,6.5 35.25,5.12 34.38,5.12 X2.17
  Bottom 0.254: v73.88,17.75 71.88,17.75 66.75,12.62 58.75,12.62 v57.88,11.75 | v38.38,6.5 38.38,7.5 v45.88,15
RB7  (via drill 0.61)
  Top 0.254: JP5.4 52,10.25 52,10.75 48.88,13.88 47.38,13.88 IC2.28 47.75,13.75 47.75,12.25 48.12,11.88 48.12,8.88 47.5,8.25 44,8.25 42.38,9.88 v36.62,9.88 | v78.62,16.88 80,15.5 R22.1 | v68.88,10.75 65.88,7.75 65.88,4.62 64.25,3 59.25,3 v54.88,7.38
  Bottom 0.254: v78.62,16.88 75.75,16.88 69.62,10.75 v68.88,10.75 | v54.88,7.38 52.12,10.12 JP5.4 | v36.62,9.88 34.38,7.62 X2.18
RC0  (via drill 0.61)
  Top 0.254: v51,30.38 54.62,26.75 56.75,26.75 IC2.11 | v43,30.62 41.62,29.25 OK1.4 41.5,29.12 41.12,29.12 36.88,24.88 36.88,23.12 R4.1
  Bottom 0.254: v51,30.38 47.12,30.38 46.25,31.25 43.62,31.25 v43,30.62
RC1  (via drill 0.61)
  Top 0.254: v54.62,28 56.75,28 IC2.12 | OK2.4 29,29.12 30.5,27.62 v30.5,27 30.5,26.12 29.75,25.38 26.75,25.38 24.5,23.12 24.25,23.12 R5.1
  Bottom 0.254: v54.62,28 51.38,31.25 47,31.25 46.5,31.75 35.25,31.75 v30.5,27
RC2  (via drill 0.61)
  Top 0.254: v63.88,32.88 63.62,33.12 61.12,33.12 61,33 61,32.5 57.75,29.25 56.88,29.25 IC2.13 | v59,38 56.38,38 55.12,39.25 55.12,39.75 54.38,40.5 46.5,40.5 44.62,38.62 41.75,38.62 39.38,41 31.75,41 v29.5,38.75 | v17.38,30.75 17.38,30.38 16.25,29.25 OK3.4 | v14.25,25.12 13.88,25.12 11.88,23.12 11.5,23.12 R6.1
  Bottom 0.254: v63.88,32.88 63.88,33.12 v59,38 | v29.5,38.75 25.62,34.88 18.62,34.88 17.38,33.62 v17.38,30.75 17.38,25.25 15.75,23.62 15,23.62 14.25,24.38 v14.25,25.12
RC4  (via drill 0.61)
  Top 0.254: v45.88,30.38 47.25,30.38 IC2.15 | v52.5,23.75 v49.38,26.88 | v58.25,21.25 59.12,20.38 v59.12,8.5 | v79.25,18.75 82.5,15.5 R23.1
  Bottom 0.254: v49.38,26.88 v45.88,30.38 | v52.5,23.75 55.75,23.75 v58.25,21.25 | X2.19 36.88,5 39.5,2.38 53.38,2.38 59.12,8.12 v59.12,8.5 59.25,8.5 60,9.25 63.12,9.25 66,12.12 69.5,12.12 74.75,17.38 74.75,17.88 75.62,18.75 v79.25,18.75
RC5  (via drill 0.61)
  Top 0.254: v55.5,25.12 51.5,29.12 47.38,29.12 IC2.16 | v70.38,19.88 80.62,19.88 85,15.5 R24.1 84.88,15.5 83.62,14.25 61.75,14.25 60.25,12.75 v60.25,7.12 | v50,4.25 45.5,4.25 42.25,7.5 36.88,7.5 X2.20 | v52.5,4.25 56.62,4.25 v57,3.88
  Bottom 0.254: v55.5,25.12 65.12,25.12 v70.38,19.88 | v52.5,4.25 v50,4.25 | v60.25,7.12 v57,3.88
RC6  (via drill 0.61)
  Top 0.254: v52.25,27.12 51.5,27.88 47.38,27.88 IC2.17 | v60.12,34.12 60.12,34.5 62,36.38 v67,36.38 | v81.62,26.88 81.62,30.62 81.5,30.75 81.5,32.75 81.75,33 85.62,33 86.12,32.5 IC3.3 | v83.75,19.62 86.38,17 86.38,11.62 83.75,9 77.25,9 76.38,8.12 76.38,4.88 74,2.5 53.5,2.5 R25.2
  Bottom 0.254: v52.25,27.12 55,27.12 59.25,31.38 59.25,33.25 v60.12,34.12 | v67,36.38 72.5,36.38 81.62,27.25 v81.62,26.88 81.62,26.75 83.75,24.62 v83.75,19.62
RC7  (via drill 0.61)
  Top 0.254: v45.88,26.62 47.25,26.62 IC2.18 | v48.75,23.75 49.38,23.75 51.38,21.75 51.38,14.62 v52.5,13.5 | v87.62,29.25 87.62,32.62 86.62,33.62 86.25,33.62 IC3.2 | v86.5,22.5 80.5,22.5 80.38,22.38 75.12,22.38 v75,22.5
  Bottom 0.254: v48.75,23.75 47.94,24.56 | 47.94,24.56 v45.88,26.62 | v52.5,13.5 52.5,13 50.88,11.38 50.88,6.38 JP6.3 | v87.62,29.25 87.62,23.62 v86.5,22.5 | v75,22.5 70.62,18.12 68.62,18.12 66.5,20.25 66.5,22.62 64.88,24.25 53.25,24.25 52.88,24.62 48,24.62 47.94,24.56
SEG-A
  Top 0.254: R15.2 62.12,12.5 62.12,9.12 61.12,8.12 61.12,6.12 62.12,5.12 X3.1
SEG-B
  Top 0.254: R16.2 64.75,12.5 64.75,10.12 62.25,7.62 X3.2
SEG-C
  Top 0.254: R17.2 67.25,12.5 67.25,11.75 63.62,8.12 63.62,6.25 64.75,5.12 X3.3
SEG-D  (via drill 0.61)
  Top 0.254: v68.38,9 69.75,10.38 69.75,12.5 R18.2
  Bottom 0.254: v68.38,9 68.38,8.12 68.5,8 68.5,7.25 67.75,6.5 65.88,6.5 64.88,7.5 X3.4
SEG-E
  Top 0.254: R19.2 72.38,12.5 72.38,11.75 68.5,7.88 68.5,6.25 67.38,5.12 X3.5
SEG-F  (via drill 0.61)
  Top 0.254: v71.62,9.25 74.88,12.5 R20.2
  Bottom 0.254: v71.62,9.25 69.38,9.25 68.75,9.88 68,9.88 67.38,9.25 67.38,7.62 X3.6
SEG-G  (via drill 0.61)
  Top 0.254: v73.5,9 73.62,9 77.12,12.5 77.38,12.5 R21.2
  Bottom 0.254: v73.5,9 73.5,7.12 72.62,6.25 71,6.25 69.88,5.12 X3.7
TECKY
  Top 0.254: R22.2 80,12.5 79.62,12.5 75.88,8.75 74.5,8.75 73.5,7.75 73.5,6.12 72.5,5.12 X3.9

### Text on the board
Bottom: v1.0 | B-0051 | Stopky v1.5 Final | www.sakul.cz
tPlace: B-0051 | 1 | Stopky v1.5 Final | www.sakul.cz | 1 | BT | PREVODNIK | DISPLAY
